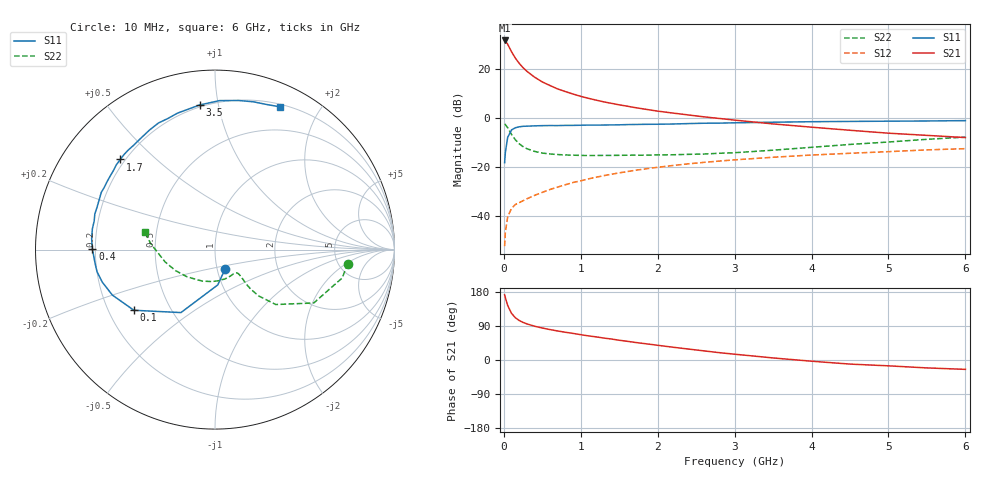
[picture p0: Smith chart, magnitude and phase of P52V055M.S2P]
! SIEMENS Small Signal Semiconductors
! BFP183
! Si NPN RF Bipolar Junction Transistor in SOT143
! VCE = 2 V  IC = 55 mA
! Common Emitter S-Parameters:  March  1996
# GHz  S  MA  R  50
!  f  S11  S21  S12  S22
! GHz  MAG  ANG  MAG  ANG  MAG  ANG  MAG  ANG
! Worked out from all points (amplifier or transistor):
!   36 points, 10 MHz to 6 GHz, reference 50 ohm
!   highest |S21| = 31.5 dB at 10 MHz (marker M1)
!   |S21| within 3 dB of that: start of sweep to 73.63 MHz
!   unconditionally stable (mu >= 1): start of sweep to 31.21 MHz; 191.2 MHz to end of sweep
!   at 250 MHz: K = 1.15, MAG = 24.8 dB, |S12| = -33.9 dB
!   at 1.4 GHz: K = 1.69, MAG = 9.6 dB, |S12| = -23.0 dB
!   at 6 GHz: K = 1.29, MAG = -1.0 dB, |S12| = -12.6 dB
!   S11 on the Smith chart (normalised r, x): 10 MHz: 1.09, -0.24; 100 MHz: 0.31, -0.30; 400 MHz: 0.19, +0.00; 1.7 GHz: 0.18, +0.39; 3.5 GHz: 0.19, +0.88; 6 GHz: 0.23, +1.53
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0.01  0.1209 -62.0  37.72 172.0  0.0024 63.2  0.7441 -6.0
0.02  0.1973 -85.5  37.1 164.2  0.0047 68.1  0.7259 -12.6
0.05  0.3989 -118.4  31.56 143.8  0.0095 61.5  0.6254 -28.4
0.1  0.5643 -143.2  22.16 123.0  0.0142 49.0  0.4565 -42.1
0.15  0.6255 -156.1  16.42 111.5  0.017 46.6  0.3545 -46.7
0.2  0.6536 -163.9  12.86 104.2  0.0185 47.8  0.2945 -47.9
0.25  0.6688 -169.4  10.49 99.1  0.0203 48.8  0.2577 -47.8
0.3  0.6729 -173.8  8.861 95.3  0.0222 51.4  0.2334 -46.9
0.4  0.6832 179.7  6.718 89.1  0.0261 54.1  0.2058 -46.0
0.5  0.69 174.9  5.377 84.4  0.03 56.6  0.1903 -45.8
0.6  0.693 170.4  4.539 80.3  0.0344 58.3  0.1824 -46.2
0.7  0.6917 166.7  3.869 76.6  0.0385 60.5  0.1774 -47.1
0.9  0.6983 160.2  3.043 70.2  0.0478 61.2  0.1724 -50.6
1.1  0.7093 153.3  2.492 63.6  0.0566 60.9  0.1696 -55.1
1.3  0.7105 147.9  2.108 57.9  0.0659 60.2  0.1706 -60.3
1.7  0.7285 136.4  1.616 46.6  0.0845 57.4  0.1725 -72.2
2.2  0.7455 123.7  1.244 33.7  0.1062 52.9  0.1757 -89.0
2.8  0.7765 109.6  0.968 19.4  0.1307 46.6  0.1885 -111.3
3.5  0.8105 96.0  0.748 5.4  0.1564 39.5  0.2179 -136.2
4.5  0.8411 81.0  0.555 -10.8  0.1885 28.9  0.2856 -165.9
5.5  0.8591 70.0  0.437 -20.9  0.2211 19.5  0.3631 174.0
6  0.8736 65.6  0.394 -24.7  0.2341 14.3  0.4026 165.6
